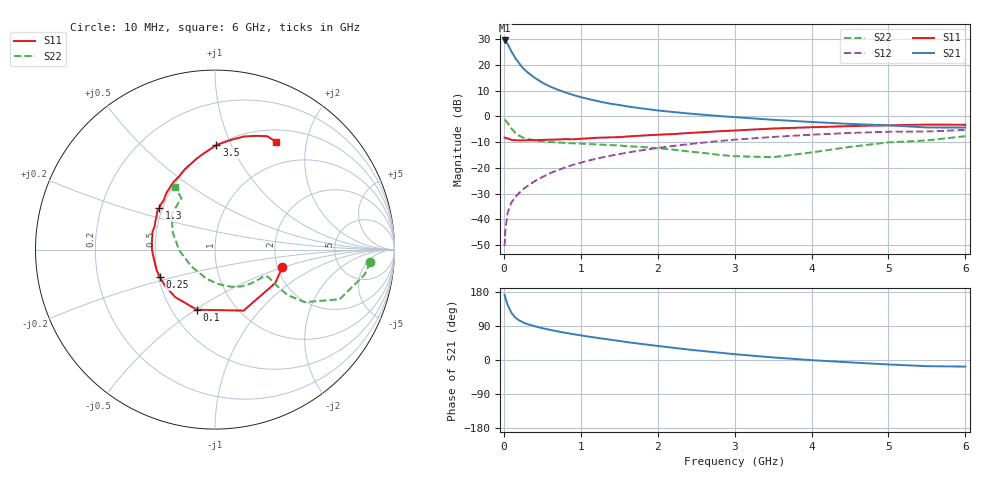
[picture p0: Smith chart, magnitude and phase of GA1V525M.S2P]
! Infineon Technologies  Discrete & RF Semiconductors
! BF775
! Si NPN RF Bipolar Junction Transistor in SOT23
! VCE = 1.5 V  IC = 25 mA
! Common Emitter S-Parameters:  May  1996
# GHz  S  MA  R  50
!  f  S11  S21  S12  S22
! GHz  MAG  ANG  MAG  ANG  MAG  ANG  MAG  ANG
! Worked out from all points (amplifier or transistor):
!   36 points, 10 MHz to 6 GHz, reference 50 ohm
!   highest |S21| = 29.6 dB at 10 MHz (marker M1)
!   |S21| within 3 dB of that: start of sweep to 76.72 MHz
!   unconditionally stable (mu >= 1): start of sweep to 12.25 MHz; 172.1 MHz to end of sweep
!   at 250 MHz: K = 1.16, MAG = 21.2 dB, |S12| = -28.4 dB
!   at 1.4 GHz: K = 1.33, MAG = 6.6 dB, |S12| = -15.2 dB
!   at 6 GHz: K = 1.08, MAG = -1.3 dB, |S12| = -5.2 dB
!   S11 on the Smith chart (normalised r, x): 10 MHz: 2.12, -0.49; 100 MHz: 0.66, -0.51; 250 MHz: 0.51, -0.18; 1.3 GHz: 0.48, +0.26; 3.5 GHz: 0.50, +0.88; 6 GHz: 0.66, +1.51
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0.01  0.3874 -14.8  30.14 171.9  0.003 84.8  0.8686 -4.7
0.02  0.3841 -29.1  29.49 164.3  0.0062 75.9  0.8427 -9.8
0.05  0.3753 -64.9  25.52 145.0  0.0136 69.9  0.7477 -21.7
0.1  0.35 -106.8  18.26 124.1  0.0214 63.5  0.5788 -30.4
0.15  0.3453 -130.0  13.68 111.8  0.0272 62.6  0.4785 -32.0
0.2  0.3437 -143.8  10.75 104.5  0.0328 64.6  0.4235 -31.1
0.25  0.3441 -153.4  8.723 99.1  0.0382 65.7  0.3872 -29.8
0.3  0.3447 -160.8  7.407 95.1  0.0437 66.9  0.3667 -28.8
0.4  0.3451 -172.1  5.683 89.2  0.0551 68.5  0.3424 -27.6
0.5  0.3509 -179.7  4.55 84.0  0.0663 69.8  0.3275 -27.2
0.6  0.3541 174.0  3.827 79.6  0.0786 70.0  0.3186 -27.7
0.8  0.3624 163.6  2.932 71.8  0.1025 69.2  0.306 -30.0
0.9  0.3596 159.3  2.626 68.3  0.1147 68.7  0.301 -31.5
1.1  0.3753 150.3  2.185 61.8  0.1384 67.1  0.2919 -35.6
1.3  0.3879 143.1  1.876 55.9  0.1626 64.7  0.2819 -39.7
1.7  0.4175 130.0  1.502 44.6  0.2092 60.0  0.2597 -49.7
2.2  0.4549 116.0  1.223 32.4  0.267 53.5  0.2267 -66.0
2.8  0.5165 101.5  1.02 19.4  0.3332 44.9  0.1789 -94.0
3.5  0.5832 89.2  0.862 6.8  0.4004 34.3  0.1617 -144.7
4.5  0.6499 75.7  0.717 -6.3  0.4778 19.4  0.2563 157.4
5.5  0.6957 65.2  0.612 -16.3  0.5107 4.6  0.3424 123.0
6  0.6903 60.4  0.61 -17.4  0.547 0.4  0.4138 123.0
